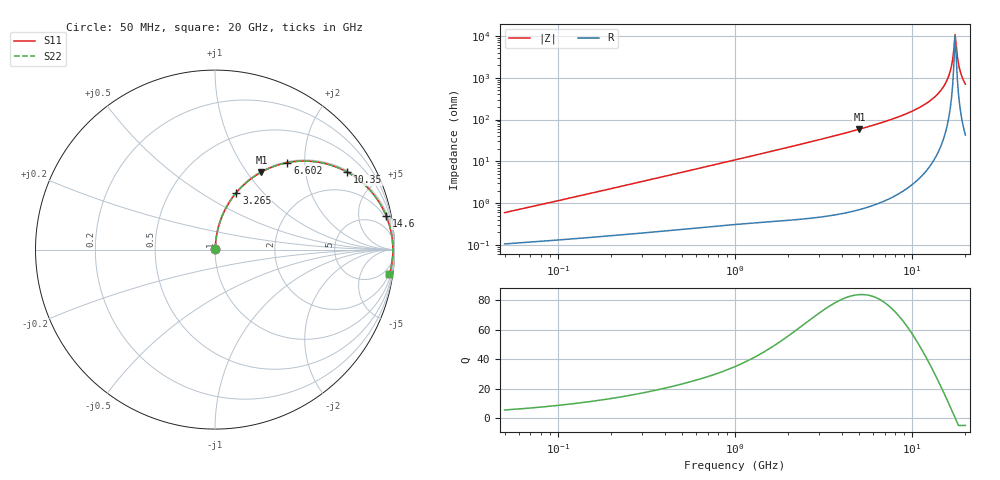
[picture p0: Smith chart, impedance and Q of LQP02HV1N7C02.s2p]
!Murata Part Number: LQP02HV1N7C02
!These Parameters are Measured in Series Mode Connection
!  o--[Z]--o
!Port1  Port2
!  o-------o
!Freq. Start=50[MHz] Stop=20[GHz], 401[Steps]
# Hz S RI R 50
!Freq.(Hz) S11(Real) S11(Imag) S21(Real) S21(Imag) S12(Real) S12(Imag) S22(Real) S22(Imag)
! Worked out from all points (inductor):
!   401 points, 50 MHz to 20 GHz, reference 50 ohm
!   read as one part in series: L = 1.84 nH near 51.52 MHz
!   highest Q = 84 at 5.041 GHz (marker M1), where L = 1.85 nH
!   self-resonance near 17.48 GHz
!   S11 on the Smith chart (normalised r, x): 50 MHz: 1.00, +0.01; 3.265 GHz: 1.01, +0.72; 6.602 GHz: 1.02, +1.64; 10.35 GHz: 1.06, +3.39; 14.6 GHz: 1, +10; 20 GHz: 2, -14
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5e7  0.00109 0.00583  0.9989 -0.00583  0.9989 -0.00583  0.00109 0.00583
1.364002e8  0.00169 0.0153  0.9983 -0.0153  0.9983 -0.0153  0.00169 0.0153
3.721004e8  0.00374 0.0405  0.9963 -0.0405  0.9963 -0.0405  0.00374 0.0405
1e9  0.0145 0.1061  0.9855 -0.1061  0.9855 -0.1061  0.0145 0.1061
2.728004e9  0.0853 0.2721  0.9147 -0.2721  0.9147 -0.2721  0.0853 0.2721
3.265178e9  0.1187 0.3168  0.8813 -0.3168  0.8813 -0.3168  0.1187 0.3168
5.041459e9  0.2586 0.4319  0.7414 -0.4319  0.7414 -0.4319  0.2586 0.4319
6.601595e9  0.4038 0.4845  0.5962 -0.4845  0.5962 -0.4845  0.4038 0.4845
7.442007e9  0.4844 0.4932  0.5156 -0.4932  0.5156 -0.4932  0.4844 0.4932
1.034674e10  0.7379 0.4307  0.2621 -0.4307  0.2621 -0.4307  0.7379 0.4307
1.257102e10  0.8776 0.3144  0.1224 -0.3144  0.1224 -0.3144  0.8776 0.3144
1.460232e10  0.9547 0.1854  0.0453 -0.1854  0.0453 -0.1854  0.9547 0.1854
1.550395e10  0.9745 0.1267  0.0255 -0.1267  0.0255 -0.1267  0.9745 0.1267
1.621653e10  0.9844 0.0808  0.0156 -0.0808  0.0156 -0.0808  0.9844 0.0808
1.670968e10  0.9886 0.0497  0.0114 -0.0497  0.0114 -0.0497  0.9886 0.0497
1.721783e10  0.9908 0.0183  0.00916 -0.0183  0.00916 -0.0183  0.9908 0.0183
1.747767e10  0.9912 0.0026  0.00879 -0.0026  0.00879 -0.0026  0.9912 0.0026
1.774144e10  0.9911 -0.0131  0.00893 0.0131  0.00893 0.0131  0.9911 -0.0131
1.800918e10  0.9904 -0.0289  0.00957 0.0289  0.00957 0.0289  0.9904 -0.0289
1.855685e10  0.9877 -0.0602  0.0123 0.0602  0.0123 0.0602  0.9877 -0.0602
1.88369e10  0.9855 -0.0758  0.0145 0.0758  0.0145 0.0758  0.9855 -0.0758
2e10  0.9722 -0.1369  0.0278 0.1369  0.0278 0.1369  0.9722 -0.1369
